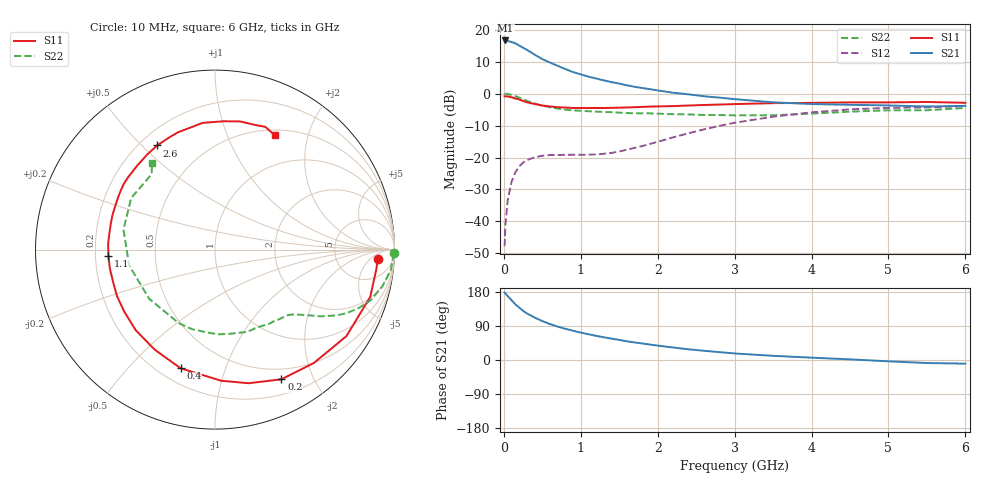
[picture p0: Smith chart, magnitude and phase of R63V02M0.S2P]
! SIEMENS Small Signal Semiconductors
! BFR193
! Si NPN RF Bipolar Junction Transistor in SOT23
! VCE = 3 V  IC = 2 mA
! Common Emitter S-Parameters:  May  1996
# GHz  S  MA  R  50
!  f  S11  S21  S12  S22
! GHz  MAG  ANG  MAG  ANG  MAG  ANG  MAG  ANG
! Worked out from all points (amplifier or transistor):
!   36 points, 10 MHz to 6 GHz, reference 50 ohm
!   highest |S21| = 16.6 dB at 20 MHz (marker M1)
!   |S21| within 3 dB of that: start of sweep to 304.7 MHz
!   unconditionally stable (mu >= 1): 1.153 GHz to 2.031 GHz
!   at 250 MHz: K = 0.24, MSG = 18.0 dB, |S12| = -21.6 dB
!   at 1.4 GHz: K = 1.11, MAG = 9.0 dB, |S12| = -18.6 dB
!   at 6 GHz: K = 0.99, MSG = 0.0 dB, |S12| = -3.9 dB
!   S11 on the Smith chart (normalised r, x): 10 MHz: 15, -9; 200 MHz: 0.37, -1.57; 400 MHz: 0.28, -0.71; 1.1 GHz: 0.25, -0.03; 2.6 GHz: 0.27, +0.56; 6 GHz: 0.57, +1.50
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0.01  0.9086 -3.4  6.653 178.1  0.0041 87.6  0.9971 -1.2
0.02  0.9057 -6.8  6.785 175.4  0.0087 85.3  0.9924 -2.6
0.05  0.9043 -16.9  6.657 168.7  0.0213 80.8  0.9858 -6.6
0.1  0.8767 -33.4  6.419 157.9  0.0418 72.0  0.9542 -12.5
0.15  0.838 -49.0  6.115 146.9  0.0586 63.8  0.9112 -18.1
0.2  0.8117 -62.9  5.652 138.2  0.0727 57.3  0.8638 -22.2
0.25  0.7677 -75.9  5.231 129.9  0.0832 51.4  0.8166 -25.6
0.3  0.7314 -87.3  4.842 122.9  0.0911 47.0  0.7713 -28.4
0.4  0.6883 -106.2  4.078 112.1  0.1007 40.2  0.6974 -32.2
0.5  0.6506 -121.2  3.463 102.6  0.1066 35.8  0.6484 -34.5
0.6  0.6297 -134.6  3.06 94.9  0.1095 33.2  0.6118 -36.5
0.7  0.6125 -145.6  2.719 88.0  0.1097 32.3  0.5826 -38.4
0.9  0.596 -161.9  2.174 77.2  0.1105 33.6  0.5458 -42.0
1.1  0.5948 -176.5  1.843 68.0  0.111 37.2  0.5304 -46.4
1.3  0.5954 171.6  1.611 60.0  0.1146 43.5  0.5159 -51.0
1.6  0.6063 156.8  1.346 49.3  0.1321 53.8  0.4977 -59.4
2.2  0.6376 132.9  1.032 33.0  0.2067 63.2  0.4766 -79.7
2.6  0.6637 119.0  0.909 24.4  0.2753 61.4  0.4627 -96.7
3.5  0.7091 95.6  0.73 11.0  0.435 46.1  0.4577 -143.3
4.5  0.7278 78.9  0.668 1.7  0.5663 25.2  0.5219 167.7
5.5  0.7391 67.7  0.628 -8.0  0.6059 6.0  0.5489 130.1
6  0.7183 62.3  0.643 -9.6  0.6398 0.7  0.5972 125.9
